FUNCTION_BLOCK Registration_CCW_DUT

VAR_IN_OUT
    SD_SMD_IO: DUT_AMCI_Stepper;
END_VAR	

VAR_INPUT
	FB_Stopping_Distance: DINT;
    FB_Programmed_Speed: UDINT;
	FB_Acceleration: UINT;
	FB_Deceleration: UINT;
	FB_Min_Registration_Distance: DINT;
	
END_VAR

VAR_OUTPUT
	Enable: BOOL :=FALSE;
	Error: BOOL :=TRUE;
END_VAR

VAR	
	I_Command_Word_1: UINT;
	D_min_registration_distance: DINT;
	
	
END_VAR

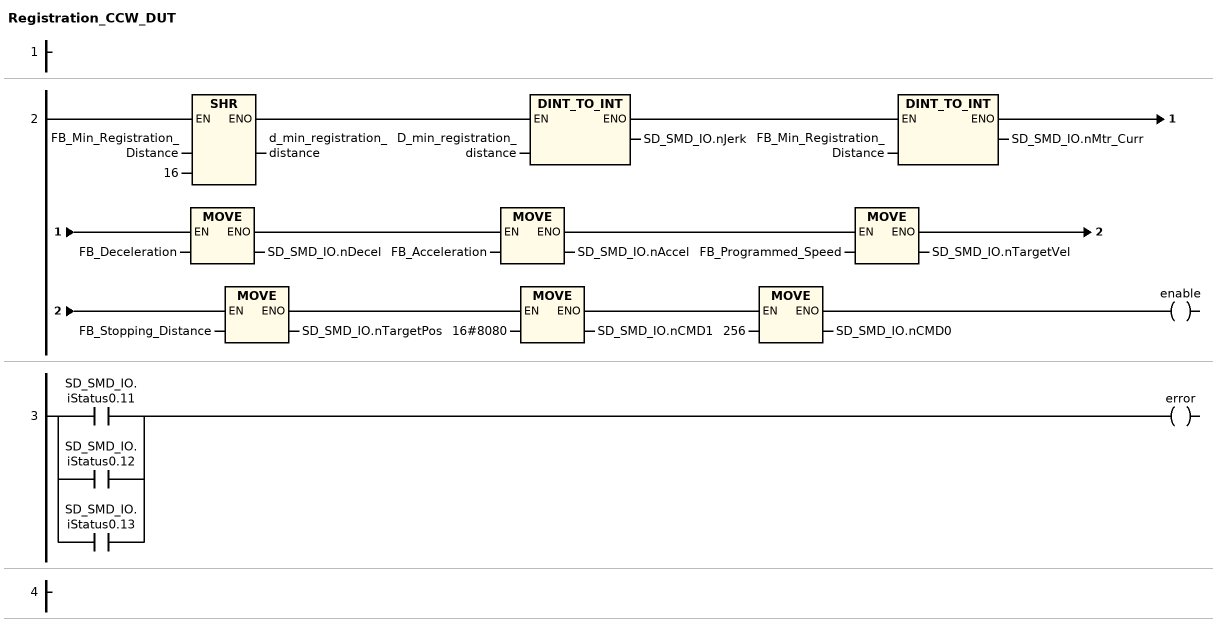
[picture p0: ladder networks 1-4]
// NETWORK 1

// NETWORK 2
d_min_registration_distance := SHR(FB_Min_Registration_Distance, 16);
SD_SMD_IO.nJerk := DINT_TO_INT(D_min_registration_distance);
SD_SMD_IO.nMtr_Curr := DINT_TO_INT(FB_Min_Registration_Distance);
SD_SMD_IO.nDecel := FB_Deceleration;
SD_SMD_IO.nAccel := FB_Acceleration;
SD_SMD_IO.nTargetVel := FB_Programmed_Speed;
SD_SMD_IO.nTargetPos := FB_Stopping_Distance;
SD_SMD_IO.nCMD1 := 16#8080;
SD_SMD_IO.nCMD0 := 256;
enable := TRUE;

// NETWORK 3
error := SD_SMD_IO.iStatus0.11 OR SD_SMD_IO.iStatus0.12 OR SD_SMD_IO.iStatus0.13;

// NETWORK 4

END_FUNCTION_BLOCK
